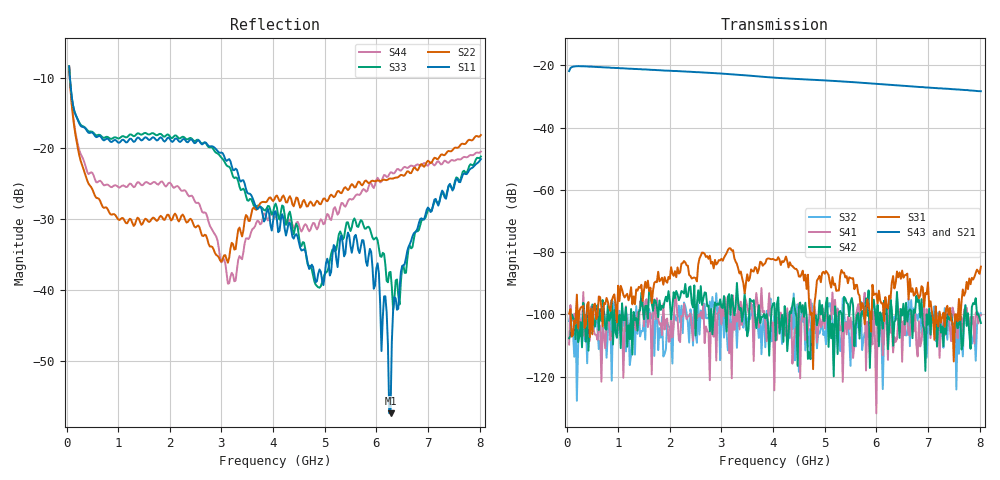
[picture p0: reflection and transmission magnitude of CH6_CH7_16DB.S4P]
!Agilent Technologies,E5071C,MY46316741,A.11.02
!Date: Mon Jun 01 10:34:56 2026
!Data & Calibration Information:
!1:CH6 INPUT 2:CH6 OUTPUT 3:CH7 INPUT 4:CH7 OUTPUT
!Freq	S11:SOLT4(ON)	S12:SOLT4(ON)	S13:SOLT4(ON)	S14:SOLT4(ON)
!	S21:SOLT4(ON)	S22:SOLT4(ON)	S23:SOLT4(ON)	S24:SOLT4(ON)
!	S31:SOLT4(ON)	S32:SOLT4(ON)	S33:SOLT4(ON)	S34:SOLT4(ON)
!	S41:SOLT4(ON)	S42:SOLT4(ON)	S43:SOLT4(ON)	S44:SOLT4(ON)
!PortZ  Port1:50+j0  Port2:50+j0  Port3:50+j0  Port4:50+j0
!Above PortZ is port z conversion or system Z0 setting when saving the data.
!When reading, reference impedance value at option line is always used.
# Hz S dB R 50
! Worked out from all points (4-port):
!   320 points, 50 MHz to 8.025 GHz, reference 50 ohm
!   strongest paths, dB at 50 MHz, 2.05 GHz, 4.05 GHz, 6.05 GHz, 8.025 GHz:
!     S43: -21.8, -21.8, -24.0, -26.0, -28.3
!     S21: -21.9, -21.8, -24.0, -25.9, -28.3
!     S31: -99.7, -86.9, -82.6, -92.4, -84.7
!     S42: -107.7, -97.6, -108.4, -110.3, -102.8
!     S41: -109.7, -107.5, -98.3, -100.0, -100.2
!     S32: -102.1, -115.8, -100.5, -99.6, -99.6
!   lowest |S11| = -57.4 dB at 6.275 GHz (marker M1), VSWR 1.00, Z = 50.1 - j0.00987 ohm
!   |S11| at or under -10 dB: 65.94 MHz to end of sweep
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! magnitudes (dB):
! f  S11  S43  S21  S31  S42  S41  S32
! 50 MHz  -8.4  -21.8  -21.9  -99.7  -107.7  -109.7  -102.1
! 700 MHz  -18.8  -20.6  -20.7  -103.9  -95.4  -104.2  -102.0
! 3.125 GHz  -21.6  -22.8  -22.8  -79.3  -94.3  -94.9  -111.6
! 5.875 GHz  -34.2  -25.8  -25.7  -99.4  -117.2  -114.3  -101.2
! 6.275 GHz  -57.4  -26.3  -26.2  -95.0  -95.3  -105.9  -98.5
! 6.625 GHz  -33.9  -26.7  -26.6  -95.2  -99.1  -106.4  -94.8
! 8.025 GHz  -21.5  -28.3  -28.3  -84.7  -102.8  -100.2  -99.6
